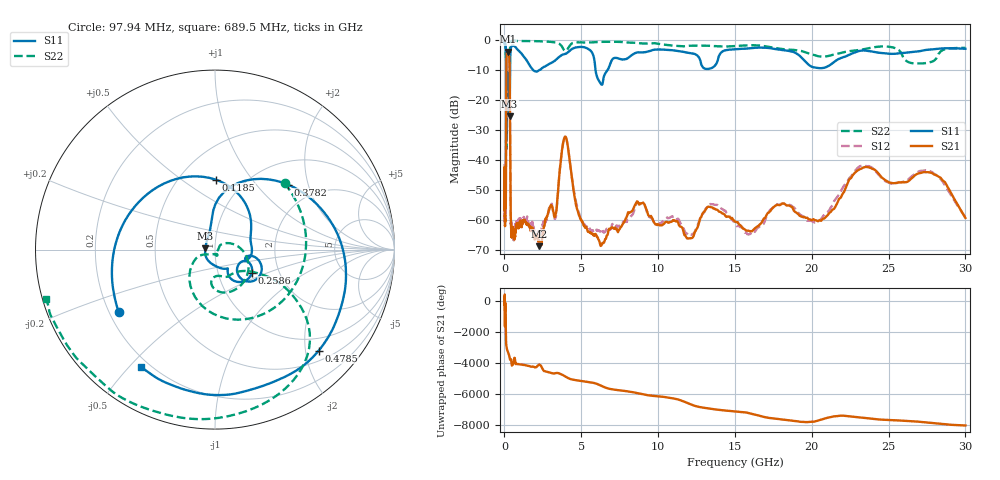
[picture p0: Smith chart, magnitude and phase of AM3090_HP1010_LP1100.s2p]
! Date/Time: Thu, Feb 28, 2019 2:04 PM
! Network Analyzer: Agilent Technologies E8364B Rev: A.07.50.67
! Sweep from 0.010 to 30.000 GHz, 1601 Points, Sweep Type: LOG
! Power Supply: 5.023 V, 0.002 A
# Hz S DB R 50
!freq MagS11 AngS11 MagS21 AngS21 MagS12 AngS12 MagS22 AngS22
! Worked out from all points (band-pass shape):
!   1601 points, 10 MHz to 30 GHz, reference 50 ohm
!   highest |S21| = -3.88 dB at 228.2 MHz (marker M1); lowest = -68.8 dB at 2.246 GHz (marker M2)
!   |S21| within 3 dB of the highest: 128.7 MHz to 324.2 MHz (195.4 MHz wide, 86.3 % of centre)
!   lowest |S11| = -25.4 dB at 333.7 MHz (marker M3), VSWR 1.11, Z = 44.9 + j0.591 ohm
!   |S11| at or under -10 dB: 122.2 MHz to 361.1 MHz (238.9 MHz wide, 98.8 % of centre); 1.864 GHz to 2.256 GHz (392 MHz wide, 19 % of centre); 5.927 GHz to 6.711 GHz (783.4 MHz wide, 12.4 % of centre)
!   |S22| runs from -36.3 to -0.1 dB; largest |S21 - S12| = 0.016
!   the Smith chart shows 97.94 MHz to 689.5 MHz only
!   S11 on the Smith chart (normalised r, x): 97.94 MHz: 0.24, -0.28; 118.5 MHz: 0.74, +0.68; 258.6 MHz: 1.45, -0.39; 378.2 MHz: 1.46, +1.50; 478.5 MHz: 0.70, -2.27; 689.5 MHz: 0.17, -0.54
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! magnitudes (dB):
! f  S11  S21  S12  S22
! 10 MHz  -0.2  -42.9  -41.3  -0.6
! 38.04 MHz  -0.5  -60.5  -60.7  -1.5
! 97.94 MHz  -3.9  -45.2  -44.0  -5.4
! 118.5 MHz  -8.2  -13.9  -13.9  -9.3
! 144.7 MHz  -14.0  -4.7  -4.7  -34.8
! 178.6 MHz  -11.9  -3.9  -3.9  -13.7
! 228.2 MHz  -16.1  -3.9  -3.8  -15.5
! 258.6 MHz  -12.3  -4.1  -4.1  -16.3
! 333.7 MHz  -25.4  -8.6  -8.6  -9.7
! 378.2 MHz  -5.3  -40.9  -41.4  -1.1
! 478.5 MHz  -1.9  -65.2  -62.1  -0.2
! 550.5 MHz  -1.9  -62.9  -65.2  -0.2
! 689.5 MHz  -2.2  -65.4  -62.7  -0.2
! 2.084 GHz  -10.5  -65.4  -65.4  -0.4
! 2.246 GHz  -10.0  -68.8  -65.0  -0.4
! 3.318 GHz  -6.7  -58.4  -59.3  -0.8
! 3.934 GHz  -4.7  -32.2  -32.3  -3.6
! 5.311 GHz  -2.6  -62.6  -62.2  -0.8
! 7.926 GHz  -6.3  -59.3  -60.6  -0.8
! 16.21 GHz  -2.6  -63.2  -63.7  -1.7
! 23.48 GHz  -3.5  -42.3  -41.9  -2.9
! 30 GHz  -2.9  -59.3  -59.1  -2.6
